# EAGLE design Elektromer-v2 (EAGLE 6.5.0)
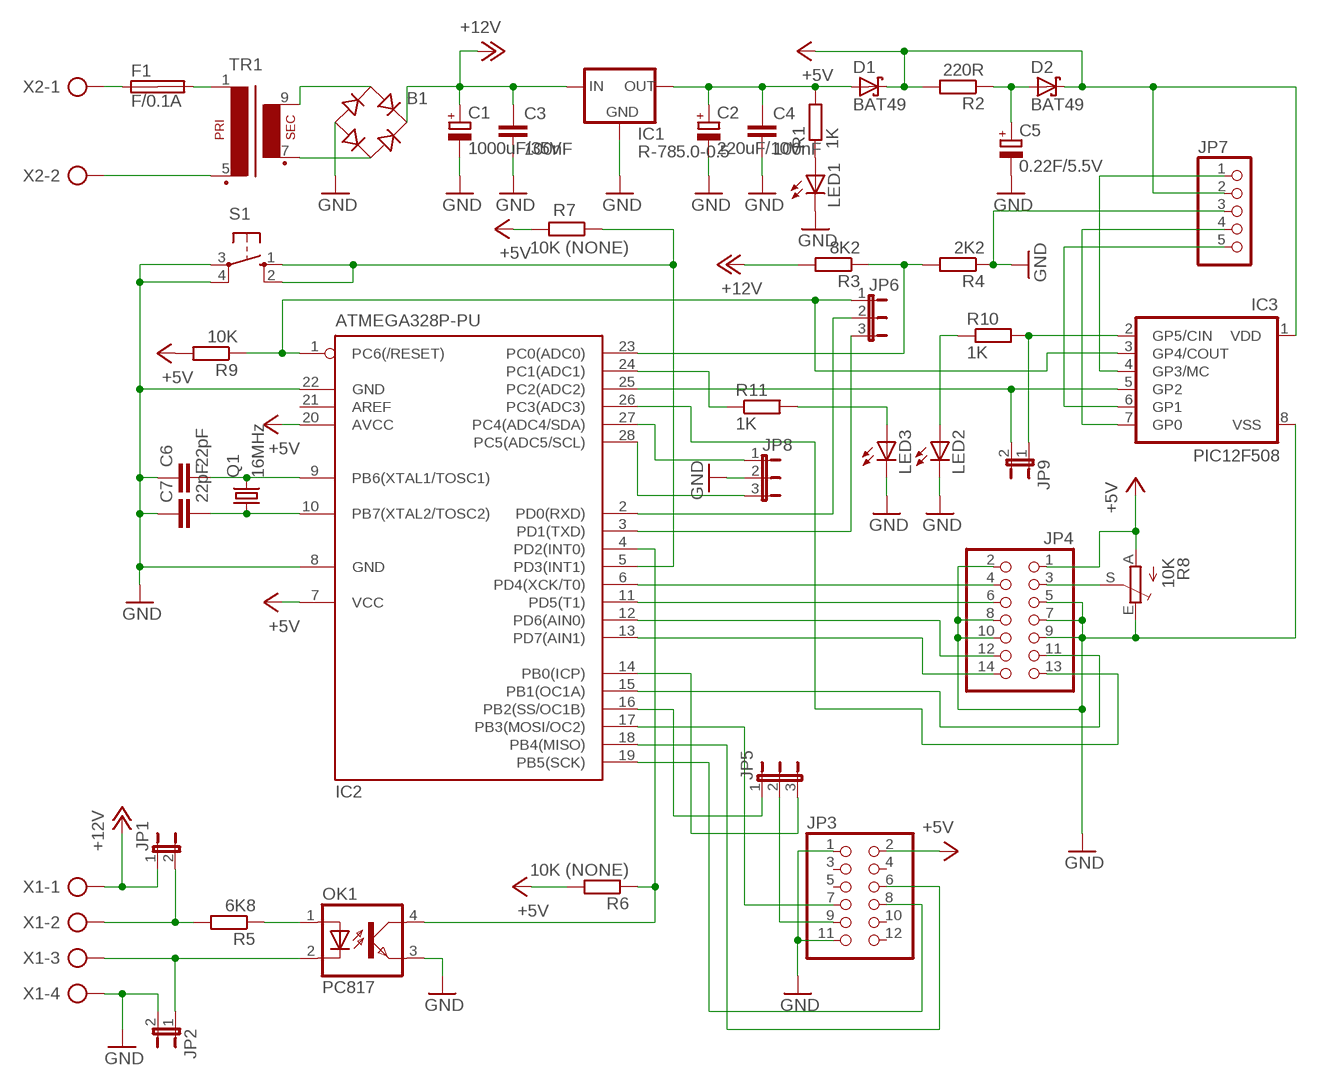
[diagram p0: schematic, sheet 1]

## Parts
B1  B-DIL  [B-DIL]
C1  1000uF/35V  CPOL-EUE5-10.5  [E5-10,5]
C2  220uF/10V  CPOL-EUE2.5-7  [E2,5-7]
C3  100nF  C-EUC025_050-024X070  [C025_050-024X070]
C4  100nF  C-EUC025_050-024X070  [C025_050-024X070]
C5  0.22F/5.5V  CPOL-EUE5-13  [E5-13]
C6  22pF  C-EUC025_050-024X070  [C025_050-024X070]
C7  22pF  C-EUC025_050-024X070  [C025_050-024X070]
D1  BAT49  [DO41-10]
D2  BAT49  [DO41-10]
F1  F/0.1A  SHK20L  [SHK20L]
IC1  R-785.0-0.5  78XXS  [78XXS]
IC2  ATMEGA328P-PU  MEGA8-P  [DIL28-3]
IC3  PIC12F508  PIC12C508P  [DIL8]
JP1  JP1E  [JP1]
JP2  JP1E  [JP1]
JP3  PINHD-2X6  [2X06]
JP4  PINHD-2X7  [2X07]
JP5  JP2E  [JP2]
JP6  JP2E  [JP2]
JP7  PINHD-1X5  [1X05]
JP8  JP2E  [JP2]
JP9  JP1E  [JP1]
LED1  LED3MM  [LED3MM]
LED2  LED3MM  [LED3MM]
LED3  LED3MM  [LED3MM]
OK1  PC817  [DIL04]
Q1  16MHz  CRYSTALHC49S  [HC49/S]
R1  1K  R-EU_0207/10  [0207/10]
R2  220R  R-EU_0207/10  [0207/10]
R3  8K2  R-EU_0207/10  [0207/10]
R4  2K2  R-EU_0207/10  [0207/10]
R5  6K8  R-EU_0207/10  [0207/10]
R6  10K (NONE)  R-EU_0207/10  [0207/10]
R7  10K (NONE)  R-EU_0207/10  [0207/10]
R8  10K  TRIM_EU-CA6V  [CA6V]
R9  10K  R-EU_0207/10  [0207/10]
R10  1K  R-EU_0207/10  [0207/10]
R11  1K  R-EU_0207/10  [0207/10]
S1  10-XX  [B3F-10XX]
TR1  EI30-1  [EI30-1]
X1  AK500/4  [AK500/4]
X2  AK500/2  [AK500/2]

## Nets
+5V: D1.C D2.C IC2.7(VCC) IC2.20(AVCC) IC3.1(VDD) JP3.2 JP4.1 JP7.2 R2.2 R6.2 R7.2 R8.A R9.2
+12V: B1.+ C1.+ C3.1 IC1.IN JP1.1 R3.2 X1.1
GND: B1.- C1.- C2.- C3.2 C4.2 C5.- C6.1 C7.1 IC1.GND IC2.8(GND) IC2.22(GND) IC3.8(VSS) JP2.2 JP3.1 JP3.11 JP4.2 JP4.5 JP4.7 JP4.8 JP4.9 JP4.10 JP7.3 JP8.2 LED1.K(C) LED2.K(C) LED3.K(C) OK1.3(EMIT) R4.1 R8.E S1.3(P) S1.4(P1) X1.4
N$1: F1.1A X2.1
N$2: TR1.5(P2) X2.2
N$3: F1.2A TR1.1
N$4: B1.AC2 TR1.7(S3)
N$5: B1.AC1 TR1.9(S4)
N$6: C2.+ C4.1 D1.A IC1.OUT R1.2
N$7: IC3.4(GP3/MC) JP7.1
N$8: LED1.A R1.1
N$9: IC3.7(GP0) JP7.4
N$10: C5.+ D2.A R2.1
N$11: IC3.6(GP1) JP7.5
N$12: C6.2 IC2.9(PB6(XTAL1/TOSC1)) Q1.2
N$13: C7.2 IC2.10(PB7(XTAL2/TOSC2)) Q1.1
N$14: IC2.25(PC2(ADC2)) IC3.5(GP2) JP9.2
N$15: IC2.23(PC0(ADC0)) R3.1 R4.2
N$16: JP1.2 R5.2 X1.2
N$17: OK1.1(A) R5.1
N$18: JP2.1 OK1.2(C) X1.3
N$19: IC2.4(PD2(INT0)) OK1.4(COL) R6.1
N$20: IC2.5(PD3(INT1)) R7.1 S1.1(S) S1.2(S1)
N$21: JP3.9 JP5.2
N$23: IC2.16(PB2(SS/OC1B)) JP5.1
N$24: IC2.14(PB0(ICP)) JP5.3
N$25: IC2.19(PB5(SCK)) JP3.8
N$26: IC2.18(PB4(MISO)) JP3.6
N$27: IC2.17(PB3(MOSI/OC2)) JP3.7
N$28: JP4.3 R8.S
N$29: IC3.2(GP5/CIN) JP9.1 R10.2
N$30: LED2.A R10.1
N$31: IC2.24(PC1(ADC1)) R11.1
N$32: IC2.6(PD4(XCK/T0)) JP4.4
N$33: IC2.11(PD5(T1)) JP4.6
N$34: IC2.12(PD6(AIN0)) JP4.12
N$35: IC2.13(PD7(AIN1)) JP4.14
N$36: IC2.15(PB1(OC1A)) JP4.11
N$37: IC2.26(PC3(ADC3)) JP4.13
N$38: IC2.1(PC6(/RESET)) IC3.3(GP4/COUT) JP6.1 R9.1
N$39: LED3.A R11.2
N$40: IC2.2(PD0(RXD)) JP6.2
N$41: IC2.3(PD1(TXD)) JP6.3
N$49: IC2.27(PC4(ADC4/SDA)) JP8.1
N$50: IC2.28(PC5(ADC5/SCL)) JP8.3
Unconnected: F1.1B F1.2B IC2.21(AREF) JP3.3 JP3.4 JP3.5 JP3.10 JP3.12

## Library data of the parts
B1 = rectifier:B-DIL: RECTIFIER
C1 C2 C5 = rcl:CPOL-EU: POLARIZED CAPACITOR, European symbol
C3 C4 C6 C7 = rcl:C-EU: CAPACITOR, European symbol
D1 D2 = diode:BAT49: DIODE
F1 = fuse:SHK20L: FUSE HOLDER 5 x 20 mm, SH contact, SHH1 Schukat, E1073 Buerklin; OC_FARNELL: unknown; OC_NEWARK: unknown
IC1 = v-reg:78XXS: VOLTAGE REGULATOR
IC2 = atmel:MEGA8-P: MICROCONTROLLER 8 Kbytes FLASH, 1 kbytes SRAM, 512 bytes EEPROM, USART, 4-channel 10 bit ADC, 2-channel 8 bit ADC Pin compatible with Atmega48, ATMega88, ATMega168 Source: avr.lbr; OC_FARNELL: unknown; OC_NEWARK: unknown
IC3 = microchip-6:PIC12C*?: MICROCONTROLLER
JP1 JP2 JP9 = jumper:JP1E: JUMPER
JP3 = pinhead:PINHD-2X6: PIN HEADER
JP4 = pinhead:PINHD-2X7: PIN HEADER
JP5 JP6 JP8 = jumper:JP2E: JUMPER
JP7 = pinhead:PINHD-1X5: PIN HEADER
LED1-LED3 = led:LED: LED
OK1 = optocoupler:PC817: SHARP OPTO COUPLER; MPN: PC817X4J000F; OC_FARNELL: 9707727; OC_NEWARK: 97K7059
Q1 = crystal:CRYSTAL: CRYSTAL; OC_FARNELL: 1667008; OC_NEWARK: unknown
R1-R7 R9-R11 = rcl:R-EU_: RESISTOR, European symbol
R8 = pot:TRIM_EU-: POTENTIOMETER
S1 = switch-omron:10-XX: OMRON SWITCH; MPN: B3F-1000; OC_FARNELL: 176432; OC_NEWARK: 36M3542
TR1 = trafo:EI30-1: TRANSFORMER 1 primary winding, 1 secondary winding ERA
X1 = con-ptr500:AK500/4: CONNECTOR; OC_FARNELL: unknown; OC_NEWARK: unknown
X2 = con-ptr500:AK500/2: CONNECTOR; OC_FARNELL: unknown; OC_NEWARK: unknown

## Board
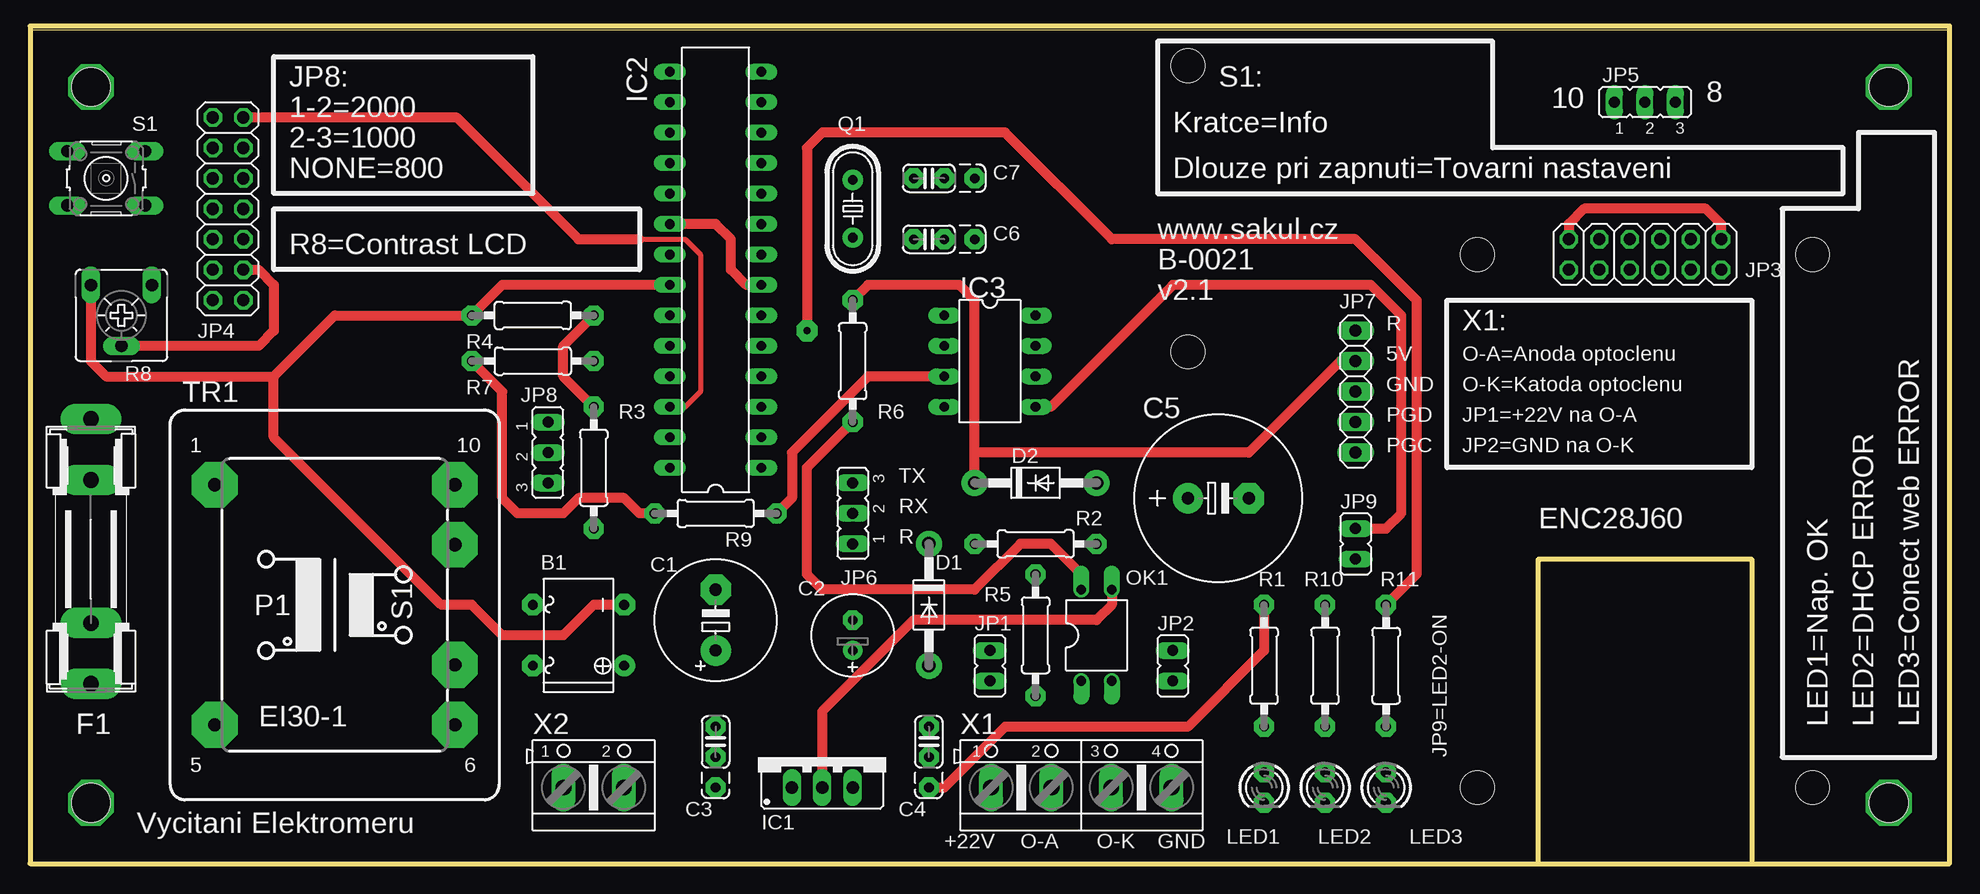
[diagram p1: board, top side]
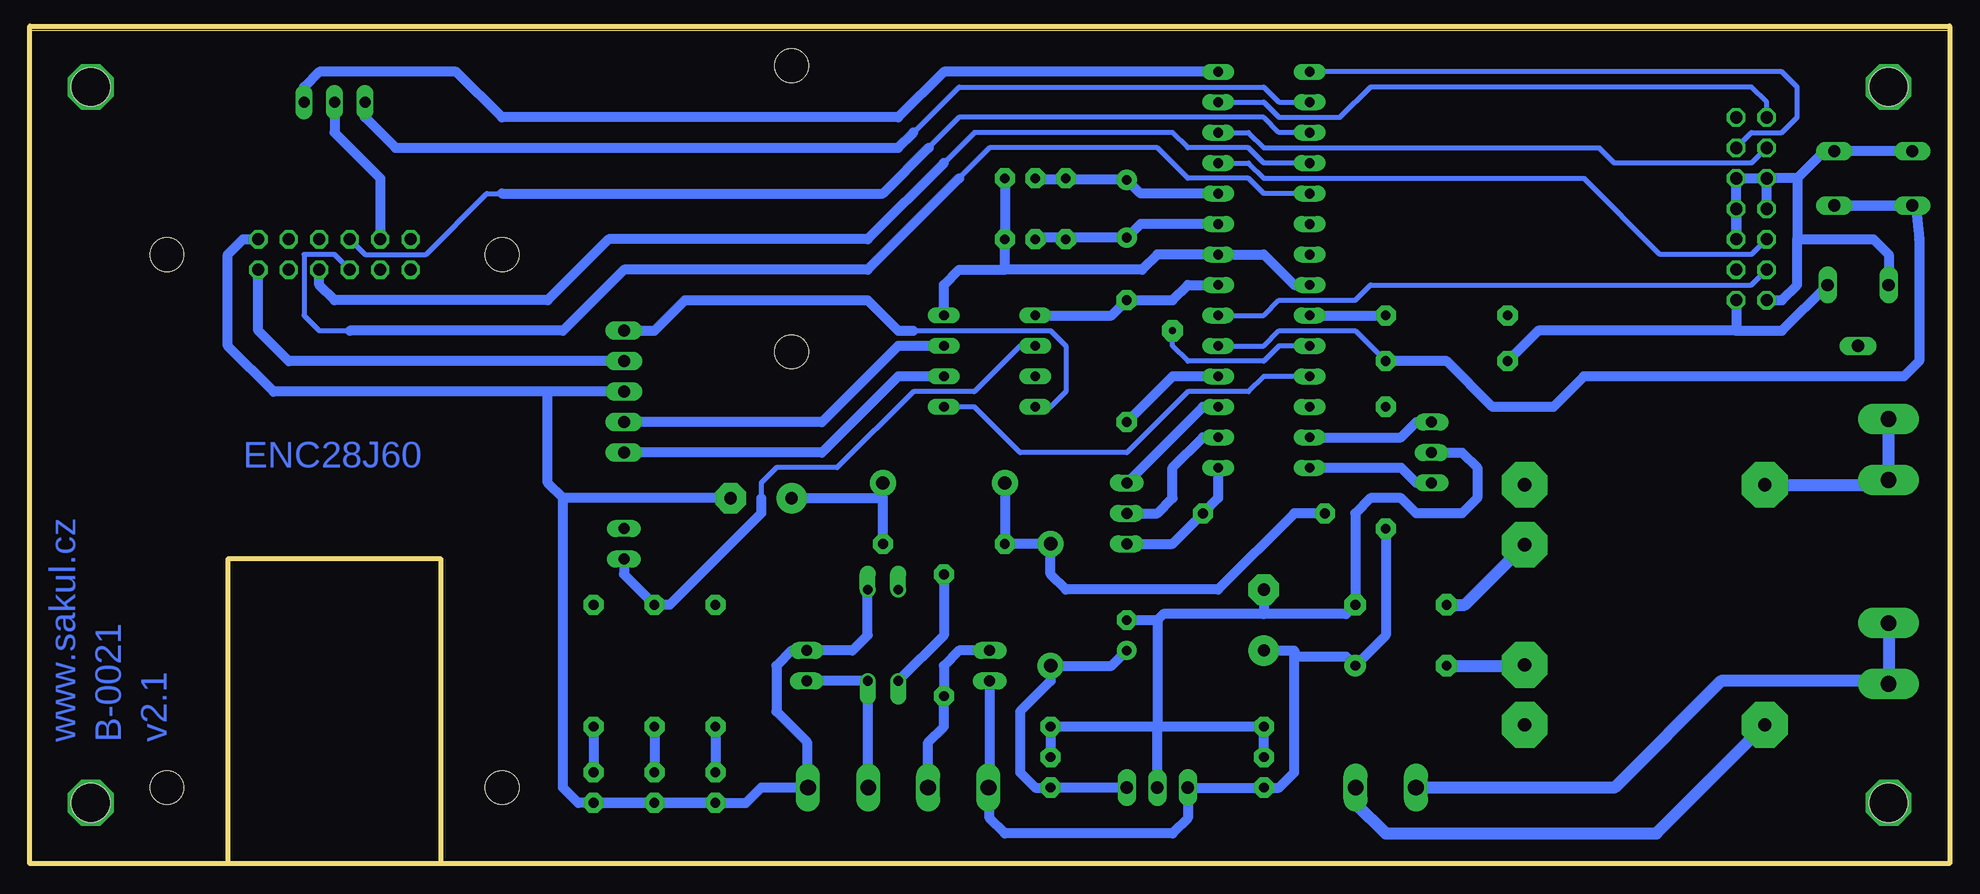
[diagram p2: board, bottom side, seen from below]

Size 160 x 69.52 mm. Coordinates in mm from the lower left corner, seen from the top.
Outline: 0,0 160,0 160,69.52 0,69.52 0,0
Copper layers (1*16): Top 0.035mm / dielectric 1.5mm / Bottom 0.035mm
Design rules "default": minimum track width 10mil, minimum drill 24mil, track to track 8mil, track to pad 8mil, pad to pad 8mil, via to via 8mil, smd to smd 8mil, copper to edge 40mil, drill to drill 8mil, minimum pad ring 10mil, minimum via ring 8mil, stop-mask expansion 4mil, vias tented up to drill 0mil, thermal gap 10mil
Holes 3.2 mm at 5.08,64.77 5.08,5.08 154.94,64.77 154.94,5.08
Holes 2.8 mm at 120.65,50.8 148.59,50.8 120.65,6.35 148.59,6.35 96.52,66.54 96.52,42.68
Milling: 9 lines

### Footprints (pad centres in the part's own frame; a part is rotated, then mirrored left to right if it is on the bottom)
B-DIL = drill 0.813 pad 1.778: + -2.54,-3.81 | drill 0.813 pad 1.778 octagon: - 2.54,-3.81; AC1 2.54,3.81; AC2 -2.54,3.81
E5-10,5 = drill 1.016 pad 2.54: + -2.54,0 | drill 1.016 pad 2.54 octagon: - 2.54,0
E2,5-7 = drill 0.813 pad 1.6: + -1.27,0 | drill 0.813 pad 1.6 octagon: - 1.27,0
C025_050-024X070 = drill 0.813 pad 1.676 octagon: 1 -3.81,0; 2 -1.27,0; 3 1.27,0
E5-13 = drill 1.016 pad 2.54: + -2.54,0 | drill 1.016 pad 2.54 octagon: - 2.54,0
DO41-10 = drill 1.118 pad 2.184: A 5.08,0; C -5.08,0
SHK20L = drill 1.321 pad 2.54 long: 1A -10.414,0; 1B -5.334,0; 2A 11.684,0; 2B 6.604,0
78XXS = drill 1.016 long: GND 0,-2.54; IN -2.54,-2.54; OUT 2.54,-2.54
DIL28-3 = drill 0.813 long: 1 -16.51,-3.81; 2 -13.97,-3.81; 3 -11.43,-3.81; 4 -8.89,-3.81; 5 -6.35,-3.81; 6 -3.81,-3.81; 7 -1.27,-3.81; 8 1.27,-3.81; 9 3.81,-3.81; 10 6.35,-3.81; 11 8.89,-3.81; 12 11.43,-3.81; 13 13.97,-3.81; 14 16.51,-3.81; 15 16.51,3.81; 16 13.97,3.81; 17 11.43,3.81; 18 8.89,3.81; 19 6.35,3.81; 20 3.81,3.81; 21 1.27,3.81; 22 -1.27,3.81; 23 -3.81,3.81; 24 -6.35,3.81; 25 -8.89,3.81; 26 -11.43,3.81; 27 -13.97,3.81; 28 -16.51,3.81
DIL8 = drill 0.813 long: 1 -3.81,-3.81; 2 -1.27,-3.81; 3 1.27,-3.81; 4 3.81,-3.81; 5 3.81,3.81; 6 1.27,3.81; 7 -1.27,3.81; 8 -3.81,3.81
JP1 = drill 0.914 long: 1 0,-1.27; 2 0,1.27
2X06 = drill 1.016 octagon: 1 -6.35,-1.27; 2 -6.35,1.27; 3 -3.81,-1.27; 4 -3.81,1.27; 5 -1.27,-1.27; 6 -1.27,1.27; 7 1.27,-1.27; 8 1.27,1.27; 9 3.81,-1.27; 10 3.81,1.27; 11 6.35,-1.27; 12 6.35,1.27
2X07 = drill 1.016 octagon: 1 -7.62,-1.27; 2 -7.62,1.27; 3 -5.08,-1.27; 4 -5.08,1.27; 5 -2.54,-1.27; 6 -2.54,1.27; 7 0,-1.27; 8 0,1.27; 9 2.54,-1.27; 10 2.54,1.27; 11 5.08,-1.27; 12 5.08,1.27; 13 7.62,-1.27; 14 7.62,1.27
JP2 = drill 0.914 long: 1 -2.54,0; 2 0,0; 3 2.54,0
1X05 = drill 1.016 long: 1 -5.08,0; 2 -2.54,0; 3 0,0; 4 2.54,0; 5 5.08,0
LED3MM = drill 0.813 pad 1.676 octagon: A -1.27,0; K 1.27,0
DIL04 = drill 0.813 offset: 1 -1.27,-3.81; 2 1.27,-3.81; 3 1.27,3.81; 4 -1.27,3.81
HC49/S = drill 0.813 pad 1.676: 1 -2.413,0; 2 2.413,0
0207/10 = drill 0.813 pad 1.676 octagon: 1 -5.08,0; 2 5.08,0
CA6V = drill 1.016 long: A -2.54,-2.54; E 2.54,-2.54; S 0,2.54
B3F-10XX = drill 1.016 long: 1 -3.251,2.261; 2 3.251,2.261; 3 -3.251,-2.261; 4 3.251,-2.261
EI30-1 = drill 1.118 pad 3.81 octagon: 1 -10.008,10.008; 5 -10.008,-10.008; 6 10.008,-10.008; 7 10.008,-5.004; 9 10.008,5.004; 10 10.008,10.008
AK500/4 = drill 1.321 long: 1 -7.518,0; 2 -2.489,0; 3 2.489,0; 4 7.518,0
AK500/2 = drill 1.321 long: 1 -2.515,0; 2 2.515,0

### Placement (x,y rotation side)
B1  45.72,19.05 90 top
C1  57.15,20.32 90 top
C2  68.58,19.05 90 top
C3  57.15,10.16 90 top
C4  74.93,10.16 90 top
C5  99.06,30.48 0 top
C6  74.93,52.07 180 top
C7  74.93,57.15 180 top
D1  74.93,21.59 270 top
D2  83.82,31.75 0 top
F1  5.08,25.4 90 top
IC1  66.04,8.89 0 top
IC2  57.15,49.53 90 top
IC3  80.01,41.91 270 top
JP1  80.01,16.51 0 top
JP2  95.25,16.51 0 top
JP3  134.62,50.8 180 top
JP4  16.51,54.61 90 top
JP5  134.62,63.5 0 top
JP6  68.58,29.21 90 top
JP7  110.49,39.37 270 top
JP8  43.18,34.29 270 top
JP9  110.49,26.67 0 top
LED1  102.87,6.35 270 top
LED2  107.95,6.35 270 top
LED3  113.03,6.35 270 top
OK1  88.9,19.05 0 top
Q1  68.58,54.61 270 top
R1  102.87,16.51 90 top
R2  83.82,26.67 180 top
R3  46.99,33.02 270 top
R4  41.91,45.72 0 top
R5  83.82,19.05 270 top
R6  68.58,41.91 90 top
R7  41.91,41.91 180 top
R8  7.62,45.72 180 top
R9  57.15,29.21 180 top
R10  107.95,16.51 90 top
R11  113.03,16.51 270 top
S1  6.35,57.15 180 top
TR1  25.4,21.59 0 top
X1  87.63,6.35 0 top
X2  46.99,6.35 0 top

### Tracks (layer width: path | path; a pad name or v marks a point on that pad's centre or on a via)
+5V
  Top 0.813: JP7.2 109.22,41.91 101.6,34.29 78.74,34.29 | D2.C 78.74,34.29 | 78.74,34.29 78.74,46.99 77.47,48.26 69.85,48.26 R6.2 | R9.2 50.8,29.21 49.53,30.48 45.72,30.48 44.45,29.21 40.64,29.21 39.37,30.48 39.37,39.37 R7.2 | IC2.7 59.69,48.26 58.42,49.53 58.42,52.07 57.15,53.34 IC2.20
  Bottom 0.813: 17.78,44.45 13.97,44.45 R8.A | JP7.2 138.43,41.91 140.97,44.45 JP3.2 | D2.C R2.2 D1.C 74.93,24.13 73.66,22.86 60.96,22.86 54.61,29.21 R9.2 | JP4.1 17.78,44.45 | 17.78,44.45 34.29,44.45 R7.2 | IC3.1 69.85,45.72 R6.2 64.77,46.99 63.5,48.26 IC2.7
+12V
  Bottom 0.813: JP1.1 80.01,6.45 X1.1 80.01,6.35 80.01,3.81 78.74,2.54 64.77,2.54 63.5,3.81 IC1.IN C3.1 55.88,6.35 54.61,7.62 54.61,17.27 | 54.61,17.27 50.29,17.27 B1.+ 46.99,19.05 R3.2 | C1.+ 54.61,17.78 54.61,17.27
GND
  Top 0.813: OK1.3 90.17,21.59 88.9,20.32 73.66,20.32 66.04,12.7 IC1.GND | R8.E 5.08,41.91 6.35,40.64 20.32,40.64 | 20.32,40.64 25.4,45.72 R4.1 39.37,48.26 IC2.22 | B1.- 46.99,21.59 44.45,19.05 39.37,19.05 36.83,21.59 34.29,21.59 20.32,35.56 20.32,40.64 | JP3.1 140.97,53.34 139.7,54.61 129.54,54.61 128.27,53.34 JP3.11
  Bottom 0.813: S1.4 S1.3 10.44,59.41 12.7,57.15 | 12.7,57.15 JP4.10 | JP4.8 JP4.10 | JP4.9 JP4.7 JP4.5 JP4.9 | JP4.2 13.97,46.99 12.7,48.26 12.7,52.07 | 78.74,49.53 67.31,49.53 66.04,50.8 IC2.8 57.15,50.8 54.61,48.26 IC2.22 | 78.74,49.53 C6.1 C7.1 | IC3.8 83.82,48.26 82.55,49.53 78.74,49.53 | C3.2 57.15,11.43 66.04,11.43 | 66.04,11.43 74.93,11.43 C4.2 | IC1.GND 66.04,11.43 | C2.- 66.04,20.32 | 66.04,20.32 66.04,11.43 | 66.04,20.32 65.53,20.83 57.15,20.83 | 95.25,6.45 95.25,10.16 97.79,12.7 97.79,16.51 96.52,17.78 JP2.2 91.44,17.78 90.17,19.05 OK1.3 | 95.25,6.45 X1.4 95.25,6.35 | LED3.K LED2.K LED1.K | LED1.K 100.33,5.08 99.06,6.35 95.25,6.35 | JP7.3 116.84,39.37 | 116.84,39.37 139.7,39.37 143.51,43.18 143.51,50.8 142.24,52.07 JP3.1 | C5.- 115.57,30.48 | 115.57,30.48 116.84,31.75 116.84,39.37 | 95.25,6.45 95.25,6.35 | LED1.K 114.3,5.08 115.57,6.35 115.57,30.48 | JP4.9 JP4.10 | 12.7,57.15 12.7,52.07 | 12.7,52.07 6.35,52.07 5.08,50.8 R8.E | JP8.2 40.64,34.29 39.37,33.02 39.37,30.48 40.64,29.21 44.45,29.21 45.72,30.48 48.26,30.48 49.53,29.21 B1.- 50.29,20.83 57.15,20.83 | C1.- 57.15,20.83
N$1
  Bottom 1.016: F1.1A 5.08,15.24 | 5.08,20.32 5.08,15.24 | 5.08,15.24 19.05,15.24 27.94,6.35 X2.1
N$2
  Bottom 1.016: X2.2 49.51,5.05 46.99,2.54 24.43,2.54 TR1.5
N$3
  Bottom 1.016: TR1.1 5.23,31.6 5.08,31.75 F1.2A
N$4
  Bottom 1.016: B1.AC2 35.48,16.51 TR1.7
N$5
  Bottom 1.016: B1.AC1 40.41,21.59 TR1.9
N$6
  Top 0.813: R1.2 102.87,17.78 96.52,11.43 81.28,11.43 76.2,6.35 C4.1
  Bottom 0.813: IC1.OUT C4.1 76.2,6.35 77.47,7.62 77.47,12.7 74.93,15.24 D1.A 69.85,16.51 C2.+
N$7
  Bottom 0.406: 86.36,44.45 74.93,44.45 73.66,43.18 73.66,39.37 74.93,38.1 IC3.4
  Bottom 0.813: JP7.1 107.95,44.45 105.41,46.99 90.17,46.99 87.63,44.45 86.36,44.45
N$8
  Bottom 0.813: R1.1 LED1.A
N$9
  Bottom 0.813: IC3.7 87.63,43.18 93.98,36.83 JP7.4
N$10
  Bottom 0.813: R2.1 88.9,30.48 | 88.9,30.48 D2.A | C5.+ 88.9,30.48
N$11
  Bottom 0.813: IC3.6 87.63,40.64 93.98,34.29 JP7.5
N$12
  Bottom 0.813: IC2.9 67.44,53.34 Q1.2 76.07,52.2 C6.2
N$13
  Bottom 0.813: IC2.10 67.44,55.88 Q1.1 76.07,57.02 C7.2
N$14
  Top 0.813: JP9.2 113.03,27.94 114.3,29.21 114.3,45.72 111.76,48.26 95.25,48.26 85.09,38.1 IC3.5
  Bottom 0.406: IC2.25 57.15,40.64 58.42,39.37 63.5,39.37 68.58,34.29 77.47,34.29 81.28,38.1 IC3.5
N$15
  Top 0.813: R3.1 44.45,40.64 44.45,43.18 R4.2
  Bottom 0.813: IC2.23 R4.2
N$16
  Bottom 0.813: JP1.2 82.55,17.78 83.82,16.51 R5.2 83.82,11.43 85.14,10.11 X1.2
N$17
  Bottom 0.813: R5.1 83.82,19.05 OK1.1
N$18
  Bottom 0.813: X1.3 90.17,6.4 OK1.2 JP2.1
N$19
  Top 0.813: OK1.4 87.63,24.13 85.09,26.67 82.55,26.67 78.74,22.86 66.04,22.86 64.77,24.13 64.77,33.02 R6.1
  Bottom 0.813: IC2.4 64.77,40.64 R6.1
N$20
  Bottom 0.406: IC2.5 57.15,43.18 55.88,44.45 49.53,44.45 R7.1
  Bottom 0.813: S1.2 S1.1 2.82,54.89 2.54,52.07 2.54,41.91 3.81,40.64 30.48,40.64 33.02,38.1 38.1,38.1 41.91,41.91 R7.1
N$21
  Bottom 0.813: JP5.2 134.62,60.96 130.81,57.15 JP3.9
N$22  (via drill 0.6 pad 3.81)
  other vias: 5.08,5.08
N$23
  Bottom 0.406: 86.36,60.96 82.55,64.77 57.15,64.77 55.88,63.5 IC2.16
  Bottom 0.813: JP5.1 132.08,62.23 129.54,59.69 87.63,59.69 86.36,60.96
N$24
  Bottom 0.813: IC2.14 83.82,66.04 87.63,62.23 120.65,62.23 124.46,66.04 135.89,66.04 137.16,64.77 JP5.3
N$25
  Bottom 0.406: IC2.19 57.15,55.88 58.42,57.15 63.5,57.15 66.04,59.69 80.01,59.69 82.55,57.15 | JP3.8 134.62,50.8 137.16,50.8 137.16,45.72 135.89,44.45 133.35,44.45
  Bottom 0.813: 82.55,57.15 90.17,49.53 110.49,49.53 115.57,44.45 133.35,44.45
N$26
  Bottom 0.406: IC2.18 57.15,58.42 58.42,59.69 63.5,59.69 64.77,60.96 81.28,60.96 83.82,58.42
  Bottom 0.813: 83.82,58.42 90.17,52.07 111.76,52.07 116.84,46.99 134.62,46.99 135.89,48.26 JP3.6
N$27
  Bottom 0.406: IC2.17 55.88,60.96 57.15,62.23 82.55,62.23 85.09,59.69 | JP3.7 132.08,50.8 127,50.8 121.92,55.88 120.65,55.88
  Bottom 0.813: 85.09,59.69 88.9,55.88 120.65,55.88
N$28
  Top 0.813: JP4.3 19.05,49.53 20.32,48.26 20.32,44.45 19.05,43.18 R8.S
N$29
  Bottom 0.406: IC3.2 77.47,43.18 81.28,39.37 86.36,39.37 92.71,33.02 97.79,33.02 99.06,31.75 99.06,30.48
  Bottom 0.813: 99.06,30.48 99.06,29.21 106.68,21.59 R10.2 110.49,24.13 JP9.1
N$30
  Bottom 0.813: R10.1 LED2.A
N$31  (via drill 0.6 pad 1.78)
  Top 0.813: v64.77,44.45 64.77,59.69 66.04,60.96 81.28,60.96 90.17,52.07 110.49,52.07 115.57,46.99 115.57,24.13 R11.1
  Bottom 0.406: IC2.24 55.88,43.18 57.15,41.91 63.5,41.91 64.77,43.18 v64.77,44.45
N$32
  Bottom 0.406: IC2.6 57.15,45.72 55.88,46.99 49.53,46.99 48.26,48.26 16.51,48.26 JP4.4
N$33
  Bottom 0.406: IC2.11 58.42,58.42 57.15,57.15 30.48,57.15 24.13,50.8 16.51,50.8 JP4.6
N$34
  Bottom 0.406: IC2.12 58.42,60.96 57.15,59.69 29.21,59.69 27.94,58.42 16.51,58.42 JP4.12
N$35
  Bottom 0.406: IC2.13 57.15,63.5 55.88,62.23 50.8,62.23 48.26,64.77 16.51,64.77 15.24,63.5 JP4.14
N$36
  Bottom 0.406: JP4.11 16.51,60.96 13.97,60.96 12.7,62.23 12.7,64.77 13.97,66.04 IC2.15
N$37
  Top 0.406: 50.8,52.07 54.61,52.07 55.88,50.8 55.88,39.37 54.61,38.1 IC2.26
  Top 0.813: JP4.13 35.56,62.23 45.72,52.07 50.8,52.07
N$38
  Top 0.813: IC3.3 69.85,40.64 63.5,34.29 63.5,30.48 R9.1
  Bottom 0.813: JP6.1 64.77,26.67 R9.1 60.96,30.48 IC2.1
N$39
  Bottom 0.813: R11.2 LED3.A
N$40
  Bottom 0.813: JP6.2 66.04,29.21 64.77,30.48 64.77,33.02 62.23,35.56 IC2.2
N$41
  Bottom 0.813: IC2.3 62.23,38.1 JP6.3
N$42  (via drill 0.6 pad 2.54)
  other vias: 120.65,6.35
N$43  (via drill 0.6 pad 2.54)
  other vias: 120.65,50.8
N$44  (via drill 0.6 pad 2.54)
  other vias: 148.59,50.8
N$45  (via drill 0.6 pad 2.54)
  other vias: 148.59,6.35
N$46  (via drill 0.6 pad 3.81)
  other vias: 154.94,5.08
N$47  (via drill 0.6 pad 3.81)
  other vias: 154.94,64.77
N$48  (via drill 0.6 pad 3.81)
  other vias: 5.08,64.77
N$49
  Bottom 0.813: IC2.27 45.72,35.56 44.45,36.83 JP8.1
N$50
  Bottom 0.813: IC2.28 45.72,33.02 44.45,31.75 JP8.3
N$51  (via drill 0.6 pad 2.54)
  other vias: 96.52,66.54
N$52  (via drill 0.6 pad 2.54)
  other vias: 96.52,42.68

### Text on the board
Bottom: ENC28J60 | v2.1 | B-0021 | www.sakul.cz
tPlace: JP8: | S1: | 10 | 8 | 1-2=2000 | Kratce=Info | 2-3=1000 | NONE=800 | Dlouze pri zapnuti=Tovarni nastaveni | www.sakul.cz | R8=Contrast LCD | B-0021 | v2.1 | R | X1: | 5V | O-A=Anoda optoclenu | GND | O-K=Katoda optoclenu | PGD | JP1=+22V na O-A | PGC | JP2=GND na O-K | TX | RX | ENC28J60 | R | LED1=Nap. OK | LED2=DHCP ERROR | LED3=Conect web ERROR | JP9=LED2-ON | Vycitani Elektromeru | +22V | O-A | O-K | GND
